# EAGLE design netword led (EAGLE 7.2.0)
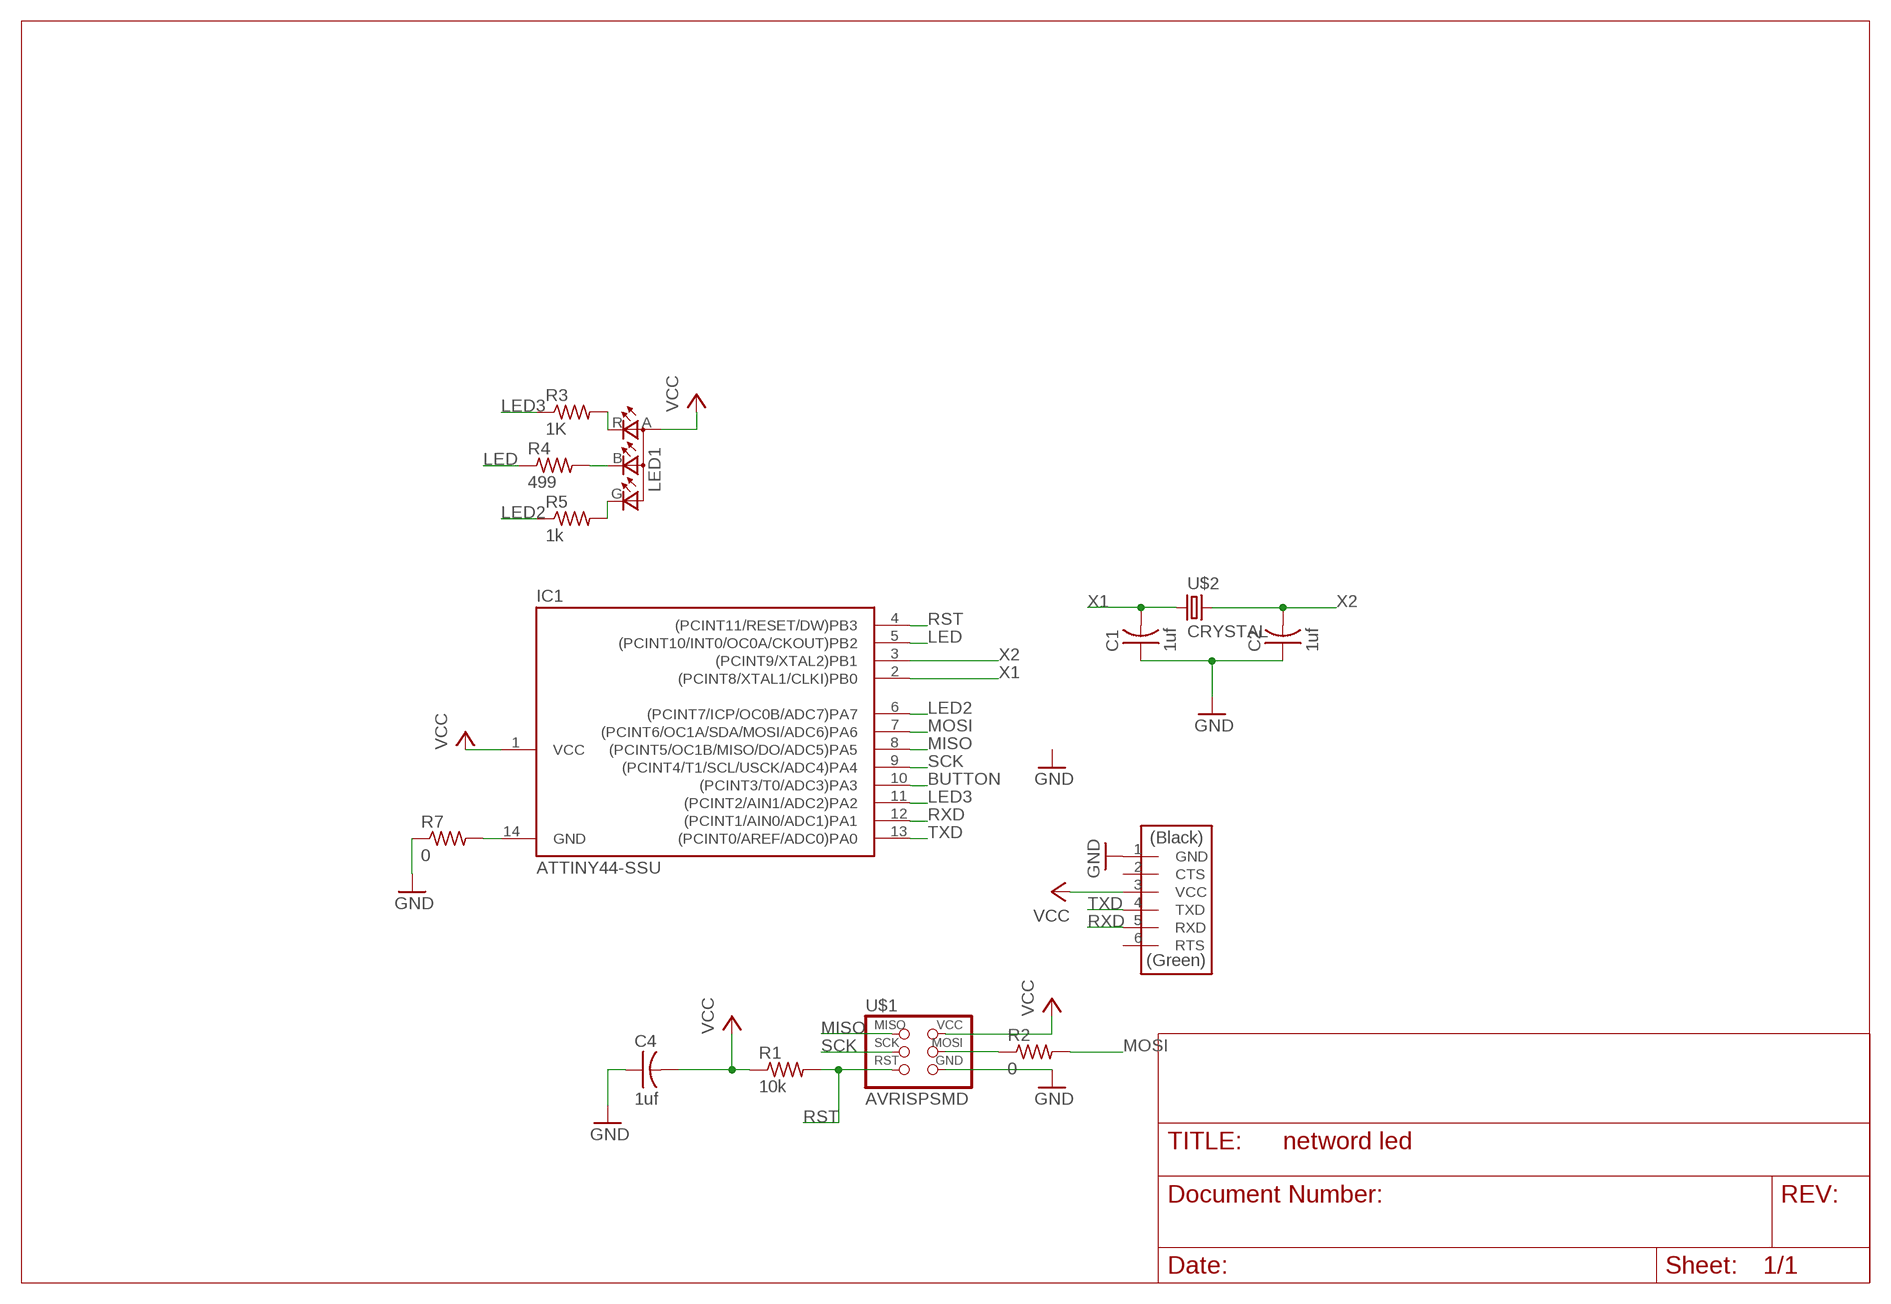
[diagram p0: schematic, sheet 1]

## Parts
C1  1uf  CAP-US1206FAB  [C1206FAB]
C2  1uf  CAP-US1206FAB  [C1206FAB]
C4  1uf  CAP-US1206FAB  [C1206FAB]
IC1  ATTINY44-SSU  [SOIC14]
LED1  LEDRGBOLD  [P-LCC-4-3]
R1  10k  RES-US1206FAB  [R1206FAB]
R2  0  RES-US1206FAB  [R1206FAB]
R3  1K  RES-US1206FAB  [R1206FAB]
R4  499  RES-US1206FAB  [R1206FAB]
R5  1k  RES-US1206FAB  [R1206FAB]
R7  0  RES-US1206FAB  [R1206FAB]
U$1  AVRISPSMD  [2X03SMD]
U$2  CRYSTAL  [2-SMD-5X3MM]
U$3  FTDI-SMD-HEADER  [1X06SMD]

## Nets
BUTTON: IC1.10((PCINT3/T0/ADC3)PA3)
GND: C1.1 C2.1 C4.1 R7.1 U$1.6(GND) U$3.1(GND)
LED: IC1.5((PCINT10/INT0/OC0A/CKOUT)PB2) R4.1
LED2: IC1.6((PCINT7/ICP/OC0B/ADC7)PA7) R5.1
LED3: IC1.11((PCINT2/AIN1/ADC2)PA2) R3.1
MISO: IC1.8((PCINT5/OC1B/MISO/DO/ADC5)PA5) U$1.1(MISO)
MOSI: IC1.7((PCINT6/OC1A/SDA/MOSI/ADC6)PA6) R2.2
N$1: R2.1 U$1.4(MOSI)
N$2: IC1.14(GND) R7.2
N$3: LED1.R(CRED) R3.2
N$4: LED1.B(CBLUE) R4.2
N$5: LED1.G(CGREEN) R5.2
RST: IC1.4((PCINT11/RESET/DW)PB3) R1.2 U$1.5(RST)
RXD: IC1.12((PCINT1/AIN0/ADC1)PA1) U$3.5(RXD)
SCK: IC1.9((PCINT4/T1/SCL/USCK/ADC4)PA4) U$1.3(SCK)
TXD: IC1.13((PCINT0/AREF/ADC0)PA0) U$3.4(TXD)
VCC: C4.2 IC1.1(VCC) LED1.A(A2) R1.1 U$1.2(VCC) U$3.3(VCC)
X1: C1.2 IC1.2((PCINT8/XTAL1/CLKI)PB0) U$2.P$1
X2: C2.2 IC1.3((PCINT9/XTAL2)PB1) U$2.P$2
Unconnected: U$3.2(CTS) U$3.6(RTS)

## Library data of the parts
C1 C2 C4 = fab:CAP-US
IC1 = fab:ATTINY44
LED1 = fab:LEDRGBOLD: OSRAM Hyper Multi TOPLED® Hyper-Bright LED LATB T686 Source: http://www.osram.convergy.de/
R1-R5 R7 = fab:RES-US: Resistor (US Symbol)
U$1 = fab:AVRISP
U$2 = 01fab:CRYSTAL
U$3 = fab:FTDI-SMD-HEADER

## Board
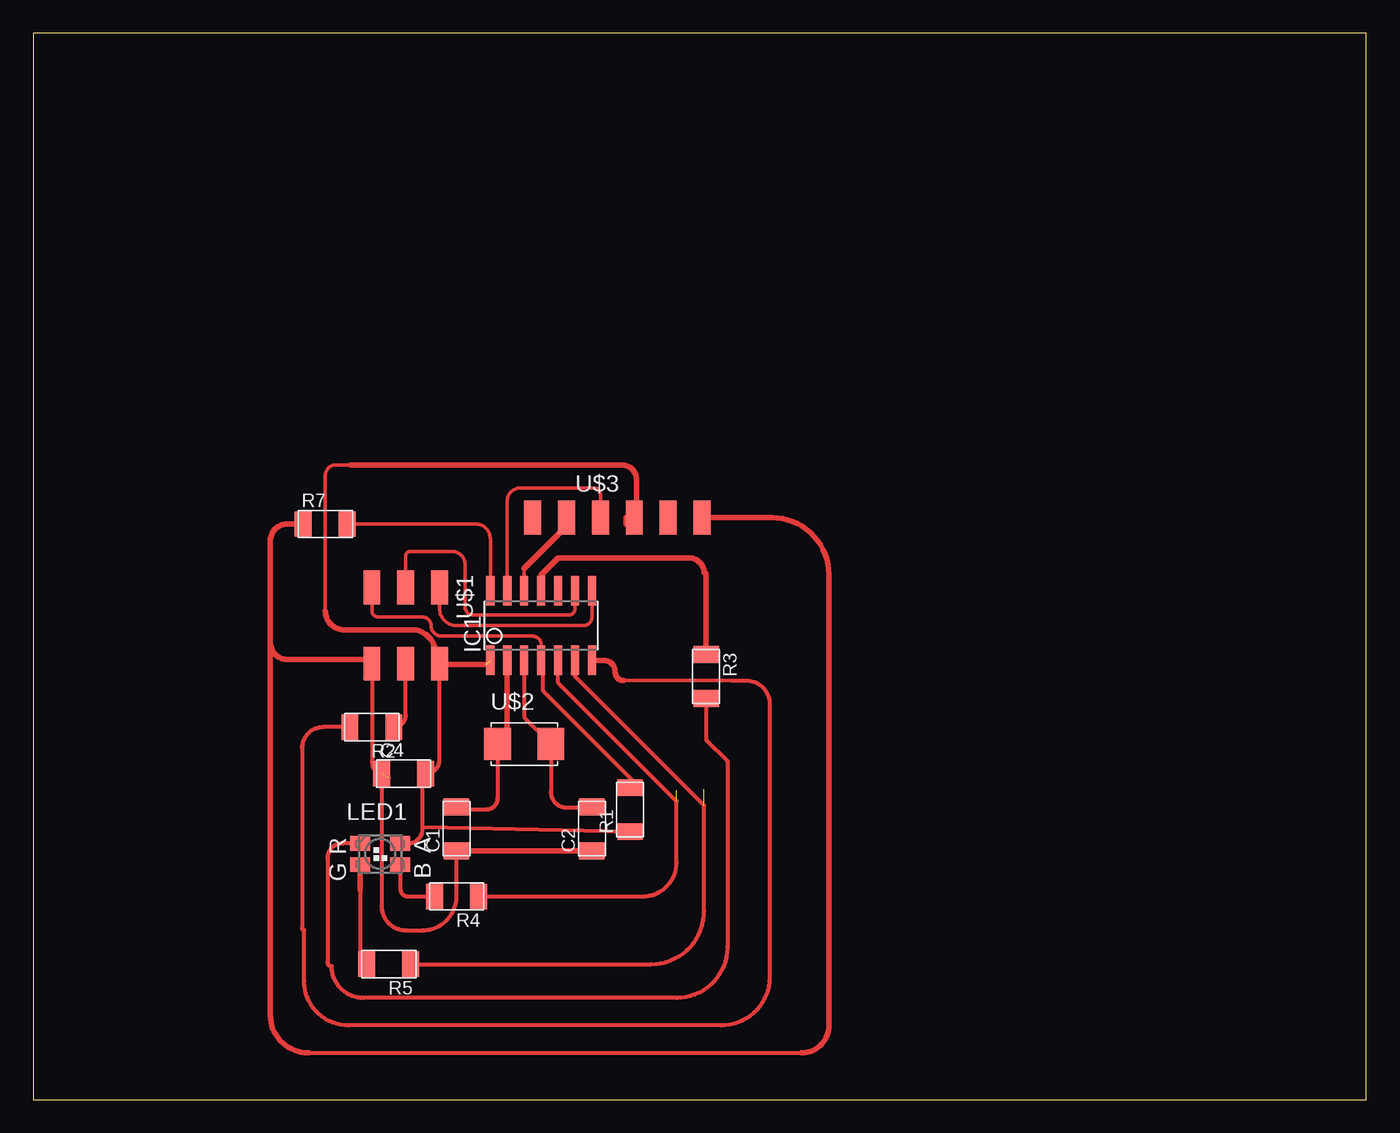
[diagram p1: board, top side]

Size 100 x 80 mm. Coordinates in mm from the lower left corner, seen from the top.
Outline: 0,0 100,0 100,80 0,80 0,0
Copper layers (1*16): Top 0.035mm / dielectric 1.5mm / Bottom 0.035mm
Design rules "default": minimum track width 10mil, minimum drill 24mil, track to track 8mil, track to pad 8mil, pad to pad 8mil, via to via 8mil, smd to smd 8mil, copper to edge 40mil, drill to drill 8mil, minimum pad ring 10mil, minimum via ring 8mil, stop-mask expansion 4mil, vias tented up to drill 0mil, thermal gap 10mil

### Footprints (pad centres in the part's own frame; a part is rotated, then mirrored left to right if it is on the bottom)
C1206FAB = smd 1.27 x 1.905: 1 -1.651,0; 2 1.651,0
SOIC14 = smd 0.61 x 2.21: 1 -3.81,-2.603; 2 -2.54,-2.603; 3 -1.27,-2.603; 4 0,-2.603; 5 1.27,-2.603; 6 2.54,-2.603; 7 3.81,-2.603; 8 3.81,2.603; 9 2.54,2.603; 10 1.27,2.603; 11 0,2.603; 12 -1.27,2.603; 13 -2.54,2.603; 14 -3.81,2.603
P-LCC-4-3 = smd 1.1 x 1.5: A -0.8,1.5; B 0.8,1.5; G 0.8,-1.5; R -0.8,-1.5
R1206FAB = smd 1.27 x 1.905: 1 -1.651,0; 2 1.651,0
2X03SMD = smd 2.54 x 1.27: 1 -2.857,2.54; 2 2.857,2.54; 3 -2.857,0; 4 2.857,0; 5 -2.857,-2.54; 6 2.857,-2.54
2-SMD-5X3MM = smd 2 x 2.4: P$1 -2,0; P$2 2,0
1X06SMD = smd 2.54 x 1.27: 1 0,6.35; 2 0,3.81; 3 0,1.27; 4 0,-1.27; 5 0,-3.81; 6 0,-6.35

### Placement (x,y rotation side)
C1  31.75,20.32 90 top
C2  41.91,20.32 90 top
C4  27.78,24.45 0 top
IC1  38.1,35.56 0 top
LED1  26.04,18.41 270 top
R1  44.77,21.75 90 top
R2  25.4,27.94 180 top
R3  50.48,31.75 270 top
R4  31.75,15.24 180 top
R5  26.67,10.16 180 top
R7  21.91,43.18 0 top
U$1  27.94,35.56 270 top
U$2  36.83,26.67 0 top
U$3  43.81,43.66 270 top

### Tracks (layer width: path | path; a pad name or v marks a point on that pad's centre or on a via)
GND  (1 unrouted)
  Top 0.254: 59.69,20.32 59.69,22.7 | 19.05,43.18 arc90 17.78,41.91
  Top 0.305: C4.1 26.13,14.51 arc90 27.94,12.7 29.21,12.7 arc90 31.75,15.24 C1.1 | 20.64,3.49 57.63,3.49 arc90 59.69,5.56 59.69,22.7 | 25.4,31.75 25.4,25.4 arc90 26.67,24.13
  Top 0.406: C2.1 C1.1 | 25.08,31.75 arc-90 25.4,32.07 | 25.4,32.07 25.4,31.75 | 25.4,32.07 U$1.6 arc90 25.08,33.02 19.05,33.02 arc-90 17.78,34.29 | U$3.1 55.4,43.66 arc-90 59.69,39.37 59.69,5.56 arc-90 57.63,3.49 | 20.64,3.49 arc-90 17.78,6.35 17.78,34.29 | R7.1 19.05,43.18 arc90 17.78,41.91 17.78,34.29
LED  (1 unrouted)
  Top 0.305: R4.1 45.72,15.24 arc90 48.26,17.78 48.26,22.38 39.37,31.27 IC1.5
LED2  (1 unrouted)
  Top 0.305: R5.1 46.35,10.16 arc90 50.32,14.13 50.32,22.07 40.64,31.75 IC1.6
LED3
  Top 0.406: IC1.11 38.1,39.37 39.37,40.64 49.21,40.64 arc-90 50.32,39.53 arc-90 50.48,39.37 R3.1
MISO
  Top 0.254: U$1.1 30.48,36.83 arc90 31.75,35.56 41.27,35.56 arc90 41.91,36.2 IC1.8
MOSI
  Top 0.254: IC1.7 41.91,33.02 | 44.29,31.43 52.39,31.43
  Top 0.305: 52.39,31.43 53.5,31.43 arc-90 55.24,29.69 55.24,9.21 arc-90 51.59,5.56 23.65,5.56 arc-90 20.32,8.89 20.32,12.7 arc-90 20.16,12.86 20.16,26.35 arc-90 21.75,27.94 R2.2
  Top 0.406: IC1.7 42.77,32.96 arc-90 43.66,32.07 arc90 44.29,31.43
N$1
  Top 0.305: 27.53,32.29 arc-90 U$1.4 27.94,28.83 arc-90 R2.1
N$2
  Top 0.254: R7.2 33.18,43.18 arc-90 34.29,42.07 IC1.14
N$3
  Top 0.305: R3.2 50.48,26.99 52.07,25.4 52.07,11.43 arc-90 48.26,7.62 24.77,7.62 arc-90 22.38,10 arc-90 22.07,10.32 22.07,18.1 arc-90 23.18,19.21 LED1.R
N$4
  Top 0.305: LED1.B 27.54,15.8 arc90 28.1,15.24 R4.2
N$5
  Top 0.305: 24.54,15.72 24.54,10.64 R5.2
  Top 0.406: 24.54,15.72 LED1.G
RST
  Top 0.254: IC1.4 38.1,34.13 arc90 37.47,34.77 30.64,34.77 arc-90 29.84,35.56 arc90 29.21,36.2 25.88,36.2 arc-90 25.4,36.67 U$1.5
  Top 0.305: R1.2 45.18,23.72 38.26,30.64 38.26,32.8 IC1.4
RXD
  Top 0.254: 36.83,39.85 IC1.12
  Top 0.406: 36.83,39.85 40.01,43.02 U$3.5
SCK
  Top 0.254: U$1.3 27.94,40.8 arc-90 28.26,41.12 31.43,41.12 arc-90 32.38,40.16 32.38,36.99 arc90 33.02,36.35 40.16,36.35 arc90 40.64,36.83 40.64,37.47 arc-90 40.8,37.62 40.8,38.01 arc90 IC1.9
TXD
  Top 0.254: IC1.13 35.56,44.93 arc-90 36.51,45.88 42.07,45.88 arc-90 42.55,45.4 U$3.4
VCC  (1 unrouted)
  Top 0.254: 21.91,36.67 21.91,46.83 arc-90 22.7,47.62 24.29,47.62
  Top 0.305: LED1.A 28.11,19.21 arc90 29.21,20.32 | 29.21,20.32 29.21,24.23 arc-90 C4.2 arc90 30.48,25.5 U$1.2 | R1.1 29.3,20.41 arc90 29.21,20.32
  Top 0.406: 33.97,32.64 30.54,32.64 arc90 U$1.2 arc-90 30.16,33.02 30.16,33.5 arc90 28.42,35.24 23.34,35.24 arc-90 21.91,36.67 | U$3.3 44.45,43.66 44.45,43.34 | 44.45,43.18 44.45,43.34 | 44.45,43.34 arc-90 45.24,44.13 45.24,46.51 arc90 44.13,47.62 24.29,47.62 23.81,47.62
X1
  Top 0.305: U$2.P$1 34.83,22.61 arc-90 33.97,21.75 31.97,21.75 arc-90 C1.2
  Top 0.406: U$2.P$1 35.56,26.67 IC1.2
X2
  Top 0.305: IC1.3 36.83,28.67 U$2.P$2 38.83,23.08 arc90 40.01,21.91 41.85,21.91 arc90 C2.2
